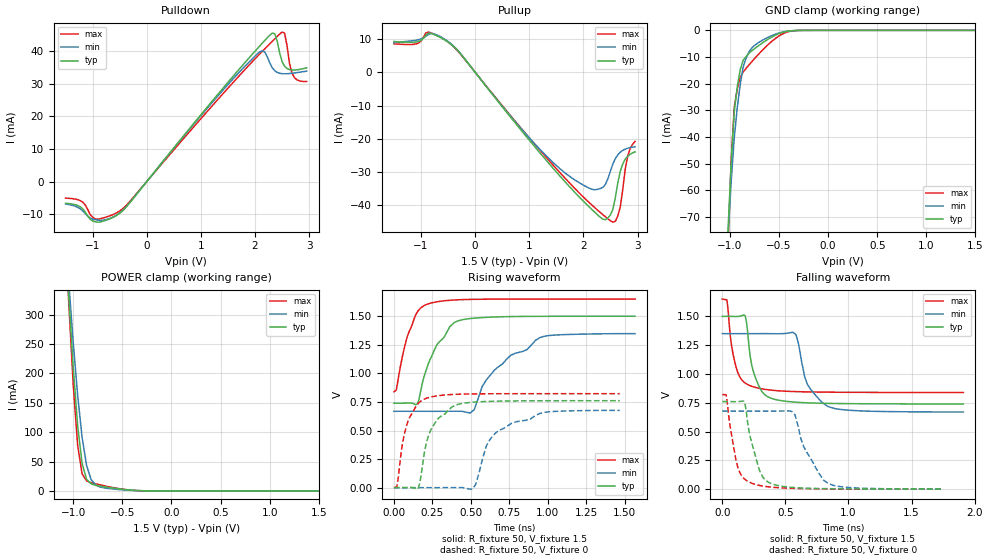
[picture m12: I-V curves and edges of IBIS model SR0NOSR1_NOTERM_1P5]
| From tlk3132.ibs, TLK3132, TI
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|   Model Cell SR0NOSR1_NOTERM_1P5
|SR0NOSR1_NOTERM_1P5
[Model]   SR0NOSR1_NOTERM_1P5
Model_type   3-state
Polarity   Non-Inverting
Enable   Active-Low
Cref =  15.0000pF
Rref =  100.0000M
Vref =  0V
Vmeas =  0.75
C_comp   1.311337p   1.240052p   1.381049p
[Temperature Range]   25   125   -40
[Voltage Range]   1.5   1.35   1.65
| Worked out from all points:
|   slope of the pulldown table from 0 to 0.225 V, typ, clamps not added: 48.2 ohm
|   slope of the pullup table from 0 to 0.225 V, typ, clamps not added: 48 ohm
|   GND clamp passes 1 mA (typ) near -0.48 V on its own axis
|   POWER clamp passes 1 mA (typ) near -0.38 V on its own axis
|   rising waveform, R_fixture 50, V_fixture 1.5: 20-80 % time 158ps typ, 314ps min, 100ps max; typ from 0.739 V to 1.5 V
|   rising waveform, R_fixture 50, V_fixture 0: 20-80 % time 110ps typ, 184ps min, 86.6ps max; typ from 0 V to 0.761 V
|   falling waveform, R_fixture 50, V_fixture 1.5: 20-80 % time 89.7ps typ, 134ps min, 76.4ps max; typ from 1.5 V to 0.74 V
|   falling waveform, R_fixture 50, V_fixture 0: 20-80 % time 102ps typ, 165ps min, 82.8ps max; typ from 0.761 V to 0.002 V
[POWER_clamp]
|   voltage   I(typ)   I(min)   I(max)
-1.5V     1.852A     1.601A     2.096A
-1.061V   377.6mA    392.9mA    374mA
-1.045V   332.8mA    356mA      321.5mA
-1.03V    292.2mA    321.8mA    275mA
-1V       211mA      253.4mA    181.9mA
-954.5mV  111.3mA    163mA      77.64mA
-909.1mV  46.83mA    91.01mA    28.92mA
-863.6mV  19.88mA    43.45mA    17.23mA
-818.2mV  12.16mA    19.6mA     14.12mA
-727.3mV  8.165mA    6.726mA    10.4mA
-409.1mV  1.376mA    880.6uA    1.274mA
1.5V      14.89nA    105.6nA    8.857nA
[Pulldown]
|   voltage   I(typ)   I(min)   I(max)
-1.5V     -6.667mA   -6.872mA   -5.079mA
-1.182V   -8.366mA   -9.005mA   -6.333mA
-954.5mV  -12.31mA   -11.68mA   -11.4mA
-454.5mV  -9.078mA   -8.982mA   -8.456mA
2.045V    40.79mA    39.16mA    38.4mA
2.182V    43.27mA    39.66mA    40.71mA
2.364V    45.32mA    33.96mA    43.74mA
2.5V      36.76mA    33.06mA    45.8mA
2.545V    35.36mA    33.02mA    45.49mA
2.682V    34.18mA    33.18mA    33.26mA
2.773V    34.24mA    33.38mA    31.19mA
2.955V    34.85mA    33.84mA    30.67mA
[Pullup]
|   voltage   I(typ)   I(min)   I(max)
-1.5V     9.208mA    8.869mA    8.526mA
-1.091V   9.066mA    9.604mA    8.486mA
-863.6mV  11.68mA    11.3mA     12.04mA
-454.5mV  8.493mA    8.644mA    8.504mA
1.727V    -34.07mA   -31.06mA   -32.95mA
2.273V    -42.98mA   -35.12mA   -41.55mA
2.409V    -44.28mA   -33.62mA   -43.43mA
2.545V    -41.14mA   -27.54mA   -45.03mA
2.636V    -33.19mA   -24.8mA    -43.12mA
2.727V    -27.53mA   -23.48mA   -35.21mA
2.818V    -25.23mA   -22.82mA   -25.22mA
2.955V    -23.93mA   -22.38mA   -20.79mA
[GND_clamp]
|   voltage   I(typ)   I(min)   I(max)
-1.5V     -1.99A     -1.518A    -2.426A
-1.015V   -72.36mA   -74.91mA   -76.76mA
-984.8mV  -48.51mA   -55.8mA    -47.87mA
-954.5mV  -30.42mA   -39.97mA   -28.58mA
-924.2mV  -21.06mA   -28.95mA   -21.99mA
-893.9mV  -14.64mA   -20.14mA   -17.66mA
-863.6mV  -11.15mA   -13.54mA   -15.57mA
-803mV    -8.521mA   -7.949mA   -12.86mA
-712.1mV  -5.867mA   -4.684mA   -9.137mA
-500mV    -1.209mA   -994.1uA   -2.074mA
-348.5mV  -89.2uA    -110.3uA   -156.7uA
1.5V      14.89nA    6.861uA    -6.796nA
[Ramp]
| variable   typ   min   max
dV/dt_f  0.4644508/89.31776p   0.4161999/0.1351671n  0.4927347/76.3115p
dV/dt_r  0.4645197/0.1083865n  0.4166215/0.1849819n  0.4991536/86.58851p
R_load = 50
[Rising Waveform]
R_fixture = 50
V_fixture = 1.5
V_fixture_min = 1.35
V_fixture_max = 1.65
|   time   V(typ)   V(min)   V(max)
0s        738.5mV    668mV      838.2mV
84ps      739.7mV    668mV      1.309V
153ps     733.5mV    668mV      1.539V
213ps     1.042V     668mV      1.603V
363ps     1.409V     668.7mV    1.639V
441ps     1.468V     668.2mV    1.645V
522ps     1.483V     683.6mV    1.648V
654ps     1.493V     1.03V      1.649V
951ps     1.499V     1.315V     1.65V
1.566ns   1.5V       1.347V     1.65V
[Rising Waveform]
R_fixture = 50
V_fixture = 0
V_fixture_min = 0
V_fixture_max = 0
|   time   V(typ)   V(min)   V(max)
0s        43.28uV    35.23uV    48.88uV
84ps      1.067mV    34.98uV    549.5mV
159ps     -1.716mV   36.56uV    738.4mV
201ps     331.4mV    39.94uV    776.6mV
276ps     585.3mV    -49.08uV   802.2mV
420ps     730.2mV    974.5uV    817.4mV
510ps     747.1mV    -12.76mV   820.1mV
621ps     754.8mV    416mV      821.4mV
765ps     758.8mV    564mV      821.8mV
1.467ns   760.7mV    675.9mV    822mV
[Falling Waveform]
R_fixture = 50
V_fixture = 1.5
V_fixture_min = 1.35
V_fixture_max = 1.65
|   time   V(typ)   V(min)   V(max)
0s        1.5V       1.35V      1.65V
36ps      1.5V       1.35V      1.643V
111ps     1.499V     1.35V      1.055V
180ps     1.507V     1.35V      923.5mV
222ps     1.15V      1.35V      898.5mV
333ps     824mV      1.35V      867.8mV
585ps     755.3mV    1.34V      847.3mV
675ps     749.9mV    910.8mV    844.9mV
840ps     745.1mV    717.1mV    842.5mV
1.911ns   740.2mV    670.7mV    839.4mV
[Falling Waveform]
R_fixture = 50
V_fixture = 0
V_fixture_min = 0
V_fixture_max = 0
|   time   V(typ)   V(min)   V(max)
0s        760.9mV    678.6mV    822.1mV
30ps      761mV      678.6mV    820.1mV
108ps     759.9mV    678.6mV    259.7mV
171ps     762.8mV    678.6mV    94.9mV
222ps     453.1mV    678.6mV    58.4mV
321ps     106.5mV    678.7mV    28.32mV
414ps     40.06mV    678.1mV    16.42mV
576ps     14.55mV    647.4mV    8.084mV
843ps     5.412mV    48.35mV    3.743mV
1.746ns   1.687mV    2.753mV    1.252mV
